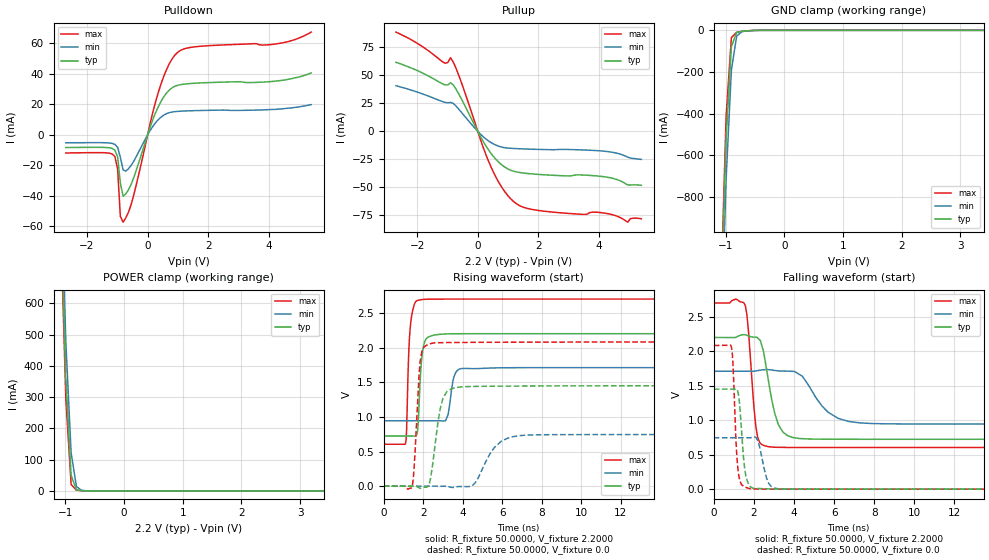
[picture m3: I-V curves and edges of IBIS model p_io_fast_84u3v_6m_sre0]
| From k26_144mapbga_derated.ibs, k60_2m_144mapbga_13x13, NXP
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[Model] p_io_fast_84u3v_6m_sre0
|   Model p_io_fast_84u3v_6m_sre0
| Library cells for typ/min/max conditions are connected as defined below:
|  pad - External Pad
|  ipp_do - Core Input
|  ipp_obe - Output Buffer Enable
|  esd_boost - vdd_s_3v
|  esd_bus - vdd_s_3v
|  ipp_ina40a_3v - NC
|  ipp_ina40b_3v - NC
|  ipp_ina_3v - NC
|  ipp_ind - NC
|  ipp_ind_3v - NC
|  vdd_s_3v - vdd_s_3v
|  vdd_s_lv - vdd_s_lv
|  vss_bulk - vss_bulk
|  vss_s_lv - vss_s_lv
| All other pins connected to ground
Model_type I/O
Polarity   Non-Inverting
Enable   Active-High
Vinl =   0.6600V
Vinh =   1.6500V
Vmeas =  1.1000V
Cref =   25.0000pF
Rref =   50.0000
Vref =   0.0V
C_comp   2.4452pF   2.2297pF   2.7119pF
[Temperature Range]   25.0000   0.1250k   -40.0000
[Voltage Range]   2.2000V   1.7100V   2.7000V
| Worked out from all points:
|   slope of the pulldown table from 0 to 0.33 V, typ, clamps not added: 18.9 ohm
|   slope of the pullup table from 0 to 0.33 V, typ, clamps not added: 21.2 ohm
|   GND clamp passes 1 mA (typ) near -0.55 V on its own axis
|   POWER clamp passes 1 mA (typ) near -0.72 V on its own axis
|   rising waveform, R_fixture 50.0000, V_fixture 2.2000: 20-80 % time 182ps typ, 243ps min, 161ps max; typ from 0.723 V to 2.2 V
|   rising waveform, R_fixture 50.0000, V_fixture 0.0: 20-80 % time 433ps typ, 918ps min, 236ps max; typ from 0 V to 1.45 V
|   falling waveform, R_fixture 50.0000, V_fixture 2.2000: 20-80 % time 594ps typ, 1.2ns min, 323ps max; typ from 2.2 V to 0.723 V
|   falling waveform, R_fixture 50.0000, V_fixture 0.0: 20-80 % time 238ps typ, 347ps min, 186ps max; typ from 1.45 V to 0 V
[Pulldown]
|Voltage   I(typ)   I(min)   I(max)
-2.7V     -8.31mA    -5.23mA    -11.88mA
-1.08V    -9.994mA   -6.23mA    -14.18mA
-990mV    -14.38mA   -8.174mA   -22.36mA
-900mV    -31.61mA   -14.63mA   -53.43mA
-810mV    -40.21mA   -22.92mA   -57.28mA
-540mV    -32.32mA   -19.93mA   -45.49mA
360mV     18.77mA    10.12mA    28.27mA
630mV     27.55mA    13.97mA    43.04mA
900mV     31.86mA    15.23mA    52.31mA
1.62V     33.93mA    15.91mA    57.87mA
4.32V     35.46mA    16.9mA     59.88mA
5.4V      40.6mA     19.8mA     67.4mA
[Pullup]
|Voltage   I(typ)   I(min)   I(max)
-2.7V     61.6mA     40.7mA     88.6mA
-1.08V    41.41mA    25.81mA    60.81mA
-900mV    43.32mA    25.75mA    65.7mA
-630mV    33.56mA    19.89mA    50.33mA
180mV     -9.091mA   -4.822mA   -14.35mA
450mV     -20.18mA   -10.26mA   -32.51mA
810mV     -30.38mA   -14.27mA   -50.71mA
1.26V     -36.2mA    -15.46mA   -64.37mA
2.25V     -38.95mA   -16.35mA   -71.56mA
4.14V     -40.49mA   -17.71mA   -72.91mA
4.95V     -47.96mA   -23.1mA    -81.2mA
5.4V      -48.23mA   -25.1mA    -78.16mA
[GND_clamp]
|Voltage   I(typ)   I(min)   I(max)
-2.7V     -21.84A    -21.72A    -21.97A
-1.08V    -1.363A    -1.529A    -1.277A
-990mV    -526.3mA   -714.4mA   -415.1mA
-900mV    -78.38mA   -191.9mA   -35.01mA
-810mV    -10.19mA   -27.77mA   -9.384mA
-720mV    -4.846mA   -5.816mA   -5.628mA
-450mV    -161.5uA   -306uA     -96.62uA
5.4V      0A         0A         0A
[POWER_clamp]
|Voltage   I(typ)   I(min)   I(max)
-2.7V     13.99A     13.91A     14.09A
-1.08V    915.5mA    1.013A     866mA
-990mV    361.3mA    476.1mA    293mA
-900mV    49.95mA    121.8mA    20.75mA
-810mV    3.622mA    14.14mA    2.341mA
-720mV    938.4uA    1.525mA    905uA
-540mV    64.25uA    64.25uA    24.86uA
5.4V      0A         0A         0A
[Ramp]
| variable   typ   min   max
dV/dt_r  0.8705/0.4332n   0.4475/0.9177n   1.2507/0.2356n
dV/dt_f  0.8860/0.5945n   0.4596/1.1997n   1.2570/0.3233n
R_load = 50.0000
[Rising Waveform]
R_fixture= 50.0000
V_fixture= 2.2000
V_fixture_min= 1.7100
V_fixture_max= 2.7000
|time   V(typ)   V(min)   V(max)
0s        723.3mV    944mV      605mV
1.111ns   723.3mV    944mV      619.6mV
1.375ns   723.4mV    944mV      2.378V
1.727ns   825.8mV    944mV      2.681V
1.913ns   1.803V     944mV      2.691V
2.141ns   2.124V     944mV      2.697V
3.133ns   2.196V     943.6mV    2.7V
3.57ns    2.199V     1.59V      2.7V
4.087ns   2.2V       1.699V     2.7V
50ns      2.2V       1.71V      2.7V
[Rising Waveform]
R_fixture= 50.0000
V_fixture= 0.0
V_fixture_min= 0.0
V_fixture_max= 0.0
|time   V(typ)   V(min)   V(max)
0s        1.4nV      47.92nV    52.08pV
1.43ns    -2.575uV   208.3nV    -15.62mV
1.536ns   179.3uV    346.6nV    242.4mV
1.84ns    -32.13mV   18.21nV    1.79V
2.468ns   291.1mV    -4.684uV   2.064V
3.005ns   1.273V     274.6uV    2.072V
4.068ns   1.435V     -6.025mV   2.074V
5.974ns   1.443V     654.2mV    2.077V
7.283ns   1.445V     737.1mV    2.079V
50ns      1.451V     745.8mV    2.084V
[Falling Waveform]
R_fixture= 50.0000
V_fixture= 2.2000
V_fixture_min= 1.7100
V_fixture_max= 2.7000
|time   V(typ)   V(min)   V(max)
0s        2.2V       1.71V      2.7V
1.575ns   2.239V     1.71V      2.663V
2.091ns   2.204V     1.715V     923.2mV
2.482ns   1.995V     1.732V     635.1mV
2.754ns   1.524V     1.733V     615.2mV
3.453ns   826mV      1.712V     605.8mV
4.641ns   728.3mV    1.544V     605.5mV
5.696ns   724.5mV    1.118V     605.2mV
7.88ns    723.4mV    952.1mV    605mV
50ns      723.3mV    944mV      605mV
[Falling Waveform]
R_fixture= 50.0000
V_fixture= 0.0
V_fixture_min= 0.0
V_fixture_max= 0.0
|time   V(typ)   V(min)   V(max)
0s        1.451V     745.8mV    2.085V
863.6ps   1.451V     745.8mV    2.075V
945.2ps   1.45V      745.8mV    1.887V
1.211ns   1.397V     745.8mV    272mV
1.536ns   308.3mV    745.5mV    34.37mV
1.838ns   32.69mV    746.1mV    6.1mV
2.206ns   8.232mV    697.4mV    2.167mV
2.726ns   4.252mV    90.23mV    126.5uV
3.343ns   960.2uV    3.378mV    71.14uV
50ns      9.103nV    54.76nV    5.189nV
